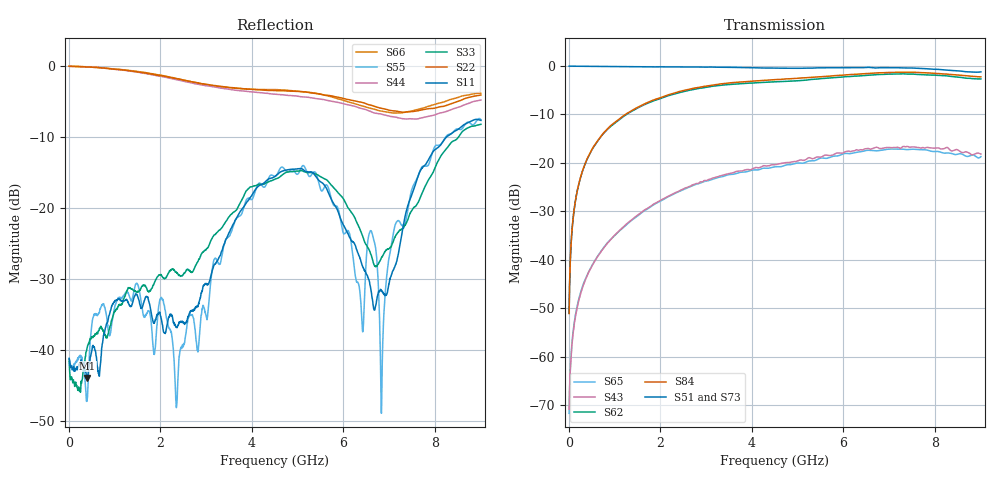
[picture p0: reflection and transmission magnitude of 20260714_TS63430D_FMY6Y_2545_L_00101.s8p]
# GHz S DB R 50
! CMT, SN0916, 25263762, 26.7.0
! Date: 15.07.2026 14:54:18
! Data: Format
! Freq S1.1:dB/Ang S1.2:dB/Ang S1.3:dB/Ang S1.4:dB/Ang S1.5:dB/Ang S1.6:dB/Ang S1.7:dB/Ang S1.8:dB/Ang
!  S2.1:dB/Ang S2.2:dB/Ang S2.3:dB/Ang S2.4:dB/Ang S2.5:dB/Ang S2.6:dB/Ang S2.7:dB/Ang S2.8:dB/Ang
!  S3.1:dB/Ang S3.2:dB/Ang S3.3:dB/Ang S3.4:dB/Ang S3.5:dB/Ang S3.6:dB/Ang S3.7:dB/Ang S3.8:dB/Ang
!  S4.1:dB/Ang S4.2:dB/Ang S4.3:dB/Ang S4.4:dB/Ang S4.5:dB/Ang S4.6:dB/Ang S4.7:dB/Ang S4.8:dB/Ang
!  S5.1:dB/Ang S5.2:dB/Ang S5.3:dB/Ang S5.4:dB/Ang S5.5:dB/Ang S5.6:dB/Ang S5.7:dB/Ang S5.8:dB/Ang
!  S6.1:dB/Ang S6.2:dB/Ang S6.3:dB/Ang S6.4:dB/Ang S6.5:dB/Ang S6.6:dB/Ang S6.7:dB/Ang S6.8:dB/Ang
!  S7.1:dB/Ang S7.2:dB/Ang S7.3:dB/Ang S7.4:dB/Ang S7.5:dB/Ang S7.6:dB/Ang S7.7:dB/Ang S7.8:dB/Ang
!  S8.1:dB/Ang S8.2:dB/Ang S8.3:dB/Ang S8.4:dB/Ang S8.5:dB/Ang S8.6:dB/Ang S8.7:dB/Ang S8.8:dB/Ang
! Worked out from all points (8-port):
!   2001 points, 10 MHz to 9 GHz, reference 50 ohm
!   strongest paths, dB at 10 MHz, 2.257 GHz, 4.505 GHz, 6.753 GHz, 9 GHz:
!     S51: -0.1, -0.2, -0.5, -0.4, -1.3
!     S73: -0.1, -0.3, -0.5, -0.5, -1.2
!     S84: -51.1, -5.8, -2.9, -1.5, -2.3
!     S62: -51.0, -6.0, -3.3, -1.8, -2.7
!     S43: -70.8, -26.5, -20.4, -16.9, -18.2
!     S65: -71.6, -26.6, -20.8, -17.5, -18.7
!   lowest |S11| = -44.0 dB at 410.1 MHz (marker M1), VSWR 1.01, Z = 50.3 - j0.575 ohm
!   |S11| at or under -10 dB: start of sweep to 8.25 GHz
